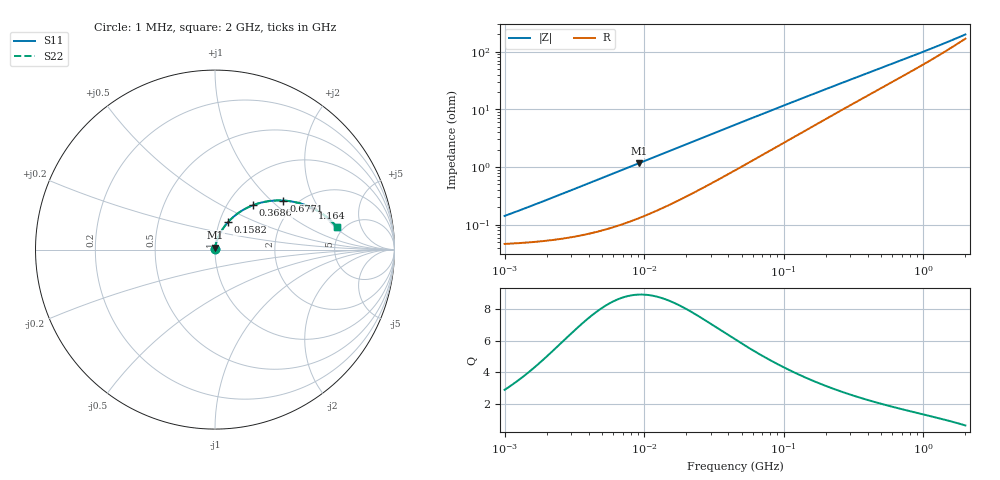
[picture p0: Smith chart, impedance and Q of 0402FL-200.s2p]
# MHz S MA R 50
!Freq  MagS11  AngS11  MagS21  AngS21  MagS12  AngS12  MagS22  AngS22
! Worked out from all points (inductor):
!   801 points, 1 MHz to 2 GHz, reference 50 ohm
!   read as one part in series: L = 21.2 nH near 1.049 MHz
!   highest Q = 8.92 at 9.15 MHz (marker M1), where L = 20.1 nH
!   S11 on the Smith chart (normalised r, x): 1 MHz: 1.00, +0.00; 158.2 MHz: 1.10, +0.35; 368.6 MHz: 1.31, +0.73; 677.1 MHz: 1.70, +1.19; 1.164 GHz: 2.48, +1.76; 2 GHz: 4.35, +2.12
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1  0.001418 70.8  0.9995 -0.1  0.9995 -0.1  0.001418 70.8
1.038736  0.001467 71.4  0.9995 -0.1  0.9995 -0.1  0.001467 71.4
1.518996  0.002074 76.1  0.9995 -0.1  0.9995 -0.1  0.002074 76.1
3.572091  0.004677 81.7  0.9993 -0.3  0.9993 -0.3  0.004677 81.7
9.150082  0.01161 82.9  0.9986 -0.7  0.9986 -0.7  0.01161 82.9
12.63918  0.01587 82.6  0.9981 -0.9  0.9981 -0.9  0.01587 82.6
25.28935  0.03097 80.6  0.9954 -1.8  0.9954 -1.8  0.03097 80.6
45.14829  0.05384 77.6  0.9898 -3.0  0.9898 -3.0  0.05384 77.6
92.06888  0.1046 71.5  0.972 -5.9  0.972 -5.9  0.1046 71.5
122.4338  0.1352 68.2  0.9581 -7.5  0.9581 -7.5  0.1352 68.2
158.2382  0.169 64.7  0.9402 -9.4  0.9402 -9.4  0.169 64.7
159.7488  0.1704 64.6  0.9395 -9.4  0.9395 -9.4  0.1704 64.6
244.9743  0.2419 57.5  0.8935 -13.2  0.8935 -13.2  0.2419 57.5
299.0698  0.2814 53.7  0.8635 -15.2  0.8635 -15.2  0.2814 53.7
368.5962  0.3265 49.4  0.8254 -17.5  0.8254 -17.5  0.3265 49.4
463.0008  0.3787 44.4  0.776 -20.0  0.776 -20.0  0.3787 44.4
565.2411  0.4259 39.9  0.7263 -22.1  0.7263 -22.1  0.4259 39.9
677.0695  0.4688 35.7  0.6768 -23.8  0.6768 -23.8  0.4688 35.7
883.4242  0.5305 29.5  0.598 -25.9  0.598 -25.9  0.5305 29.5
1163.675  0.5903 23.1  0.5121 -26.8  0.5121 -26.8  0.5903 23.1
1592.205  0.6509 15.9  0.4144 -25.5  0.4144 -25.5  0.6509 15.9
2000  0.6891 10.7  0.3474 -21.6  0.3474 -21.6  0.6891 10.7
